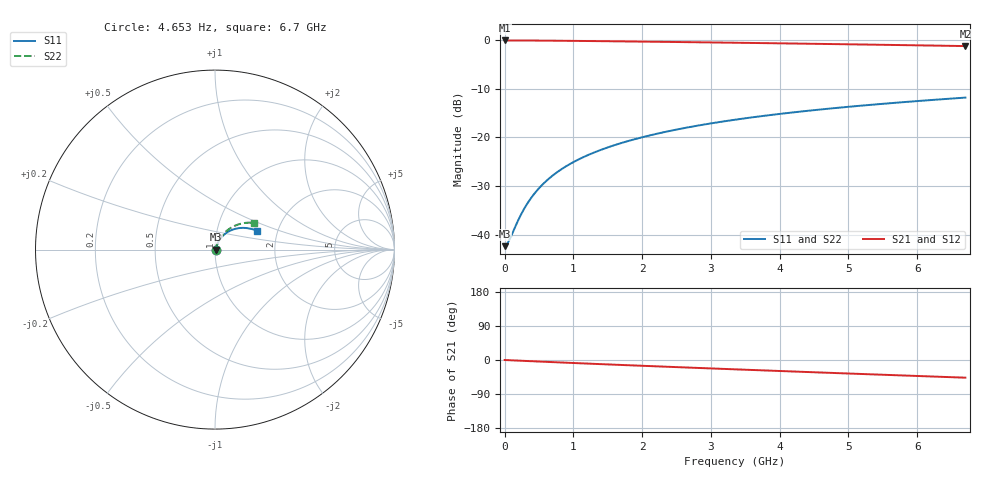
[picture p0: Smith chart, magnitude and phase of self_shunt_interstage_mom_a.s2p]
! Created Mon Jan 20 16:22:39 2014
# ghz S ma R 50
! 2 Port Network Data from data block
! freq  magS11  angS11  magS21  angS21  magS12  angS12  magS22  angS22
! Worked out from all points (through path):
!   115 points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, 4.653 Hz to 6.7 GHz, reference 50 ohm
!   highest |S21| = -0.07 dB at 4.653 Hz (marker M1); lowest = -1.2 dB at 6.7 GHz (marker M2)
!   group delay of S21, straight-line fit = 19.3 ps
!   lowest |S11| = -42.4 dB at 4.653 Hz (marker M3), VSWR 1.02, Z = 50.8 + j2.88e-08 ohm
!   |S11| at or under -10 dB: start of sweep to end of sweep
!   |S22| runs from -42.4 to -11.6 dB; largest |S21 - S12| = 0
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4.652778e-09  0.007612 0.0  0.9924 -0.0  0.9924 -0.0  0.007612 0.0
0.04652778  0.008224 19.4  0.9924 -0.4  0.9924 -0.4  0.008146 19.5
0.09305556  0.009571 34.0  0.9923 -0.8  0.9923 -0.8  0.009515 34.4
0.1861111  0.01351 51.3  0.9919 -1.5  0.9919 -1.5  0.0135 51.7
0.2326389  0.0158 56.1  0.9916 -1.9  0.9916 -1.9  0.01579 56.5
0.2791667  0.0182 59.5  0.9913 -2.3  0.9913 -2.3  0.01817 59.9
0.3722222  0.02314 63.5  0.9905 -3.0  0.9905 -3.0  0.02308 64.1
0.4885417  0.02939 65.8  0.9894 -3.9  0.9894 -3.9  0.0293 66.6
0.6048611  0.03559 66.7  0.988 -4.9  0.988 -4.9  0.03547 67.6
0.7599537  0.04367 66.7  0.986 -6.1  0.986 -6.1  0.04352 67.9
0.9538194  0.05342 65.8  0.9832 -7.6  0.9832 -7.6  0.05324 67.4
1.147685  0.06277 64.6  0.9802 -9.0  0.9802 -9.0  0.06255 66.5
1.380324  0.07352 62.9  0.9764 -10.8  0.9764 -10.8  0.07327 65.2
1.690509  0.08721 60.5  0.971 -13.0  0.971 -13.0  0.0869 63.4
2.000694  0.1003 58.1  0.9655 -15.2  0.9655 -15.2  0.09994 61.5
2.303125  0.1126 55.7  0.96 -17.4  0.96 -17.4  0.1122 59.7
2.791667  0.1315 52.0  0.951 -20.8  0.951 -20.8  0.1312 56.8
3.419792  0.1544 47.2  0.9388 -25.1  0.9388 -25.1  0.1544 53.2
3.908333  0.1712 43.6  0.929 -28.4  0.929 -28.4  0.1716 50.4
4.466667  0.1895 39.6  0.9174 -32.1  0.9174 -32.1  0.1905 47.3
5.653125  0.226 31.2  0.8919 -39.9  0.8919 -39.9  0.2289 40.7
6.7  0.2565 23.9  0.8686 -46.6  0.8686 -46.6  0.2617 34.8
